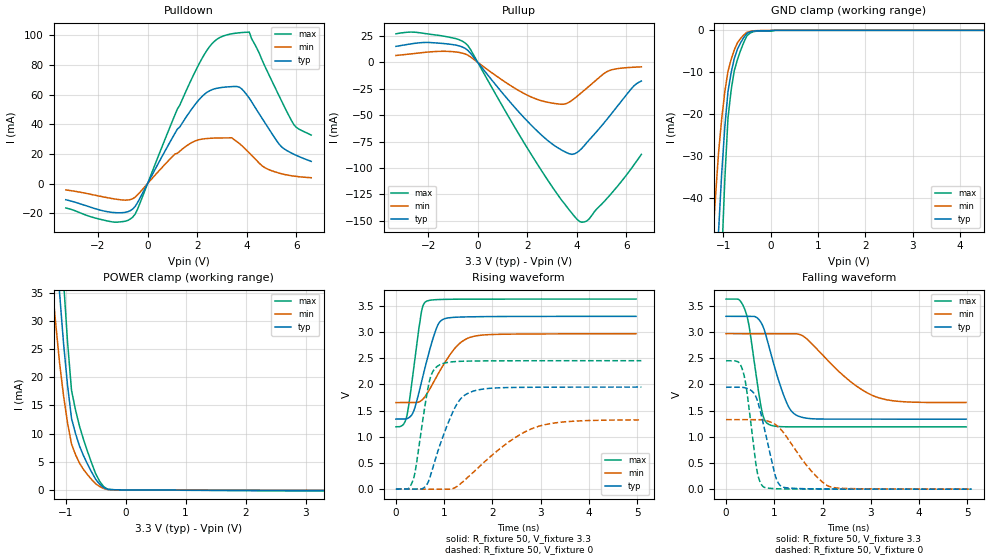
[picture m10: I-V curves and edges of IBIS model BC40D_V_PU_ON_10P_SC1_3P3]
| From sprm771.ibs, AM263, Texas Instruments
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|   Model Cell BC40D_V_PU_ON_10P_SC1_3P3
|BC40D_V_PU_ON_10P_SC1_3P3
[Model]   BC40D_V_PU_ON_10P_SC1_3P3
Model_type   I/O
Polarity   Non-Inverting
Enable   Active-Low
Vinl =  0.8V
Vinh =  2V
Cref =  15pF
Rref =  100.0000M
Vref =  0V
Vmeas =  1.65
C_comp   2.059994p   1.912853p   2.135747p
|[Input load] weak_pu_on
|[Output drive] slow
|[supplytol] 10
|[temp] ind
[Model Spec]
Vinl   0.8V   0.8V   0.8V
Vinh   2V   2V   2V
[Temperature Range]   25   125   -40
[Voltage Range]   3.3   2.97   3.63
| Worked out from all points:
|   slope of the pulldown table from 0 to 0.495 V, typ, clamps not added: 31.8 ohm
|   slope of the pullup table from 0 to 0.495 V, typ, clamps not added: 33.8 ohm
|   GND clamp passes 1 mA (typ) near -0.52 V on its own axis
|   POWER clamp passes 1 mA (typ) near -0.43 V on its own axis
|   rising waveform, R_fixture 50, V_fixture 3.3: 20-80 % time 333ps typ, 531ps min, 208ps max; typ from 1.34 V to 3.3 V
|   rising waveform, R_fixture 50, V_fixture 0: 20-80 % time 466ps typ, 1.07ns min, 244ps max; typ from 0 V to 1.95 V
|   falling waveform, R_fixture 50, V_fixture 3.3: 20-80 % time 385ps typ, 931ps min, 233ps max; typ from 3.3 V to 1.34 V
|   falling waveform, R_fixture 50, V_fixture 0: 20-80 % time 293ps typ, 644ps min, 201ps max; typ from 1.95 V to 0.002 V
| Nom Voltages:
|   VDD=1.1001, VDDS=3.3, VDDS18=1.8, ESD_BIASFET=0, VSS=0, VSSS=0
| Min Voltages:
|   VDD=0.99, VDDS=2.97, VDDS18=1.62, ESD_BIASFET=0, VSS=0, VSSS=0
| Max Voltages:
|   VDD=1.21, VDDS=3.63, VDDS18=1.98, ESD_BIASFET=0, VSS=0, VSSS=0
[POWER_clamp]
|   voltage   I(typ)   I(min)   I(max)
-3.3V     446.9mA    419.5mA    603.9mA
-1.233V   56.55mA    37.52mA    80.26mA
-1.167V   45.63mA    29.9mA     65.05mA
-1.1V     35.1mA     22.66mA    50.24mA
-1.033V   26.08mA    16.76mA    37.18mA
-966.7mV  18.62mA    11.92mA    26.33mA
-900mV    12.7mA     8.149mA    17.69mA
-833.3mV  10mA       6.265mA    14.21mA
-766.7mV  7.795mA    4.753mA    11.3mA
-566.7mV  3.199mA    1.871mA    4.823mA
-366.7mV  433.5uA    268.4uA    618.3uA
3.3V      -100.3uA   -83.23uA   -188.3uA
[Pulldown]
|   voltage   I(typ)   I(min)   I(max)
-3.3V     -10.93mA   -4.311mA   -16.48mA
-1.4V     -19.53mA   -10.23mA   -25.96mA
-600mV    -17.23mA   -10.26mA   -22.66mA
1.1V      33.82mA    19.89mA    46.25mA
2V        55.14mA    29.24mA    78.29mA
2.6V      63.35mA    30.61mA    94.45mA
3.2V      65.21mA    30.81mA    100.4mA
3.7V      65.09mA    27.02mA    101.8mA
4.1V      57.63mA    20.71mA    102.2mA
5.3V      26.68mA    7.058mA    59.31mA
5.9V      19.77mA    5.007mA    39.76mA
6.6V      14.97mA    3.923mA    32.7mA
[Pullup]
|   voltage   I(typ)   I(min)   I(max)
-3.3V     15.12mA    6.498mA    27.02mA
-1.9V     18.73mA    9.943mA    26.53mA
-900mV    16.4mA     9.888mA    22.58mA
-400mV    11.39mA    6.786mA    15.98mA
2.4V      -65.08mA   -35.06mA   -96.18mA
3.5V      -84.52mA   -39.53mA   -134mA
3.8V      -87.17mA   -36.01mA   -143mA
4.1V      -83.7mA    -30.35mA   -150.6mA
4.4V      -75.99mA   -24.42mA   -150.3mA
5.3V      -51.41mA   -7.872mA   -126.6mA
6.3V      -22.29mA   -4.606mA   -97.15mA
6.6V      -17.71mA   -4.277mA   -87.2mA
[GND_clamp]
|   voltage   I(typ)   I(min)   I(max)
-3.3V     -787.2mA   -607.8mA   -1.235A
-1.233V   -85.67mA   -52.14mA   -138.8mA
-1.167V   -66.48mA   -40.37mA   -107.8mA
-1.1V     -48.26mA   -29.37mA   -78.02mA
-1.033V   -34.3mA    -21.2mA    -54.63mA
-966.7mV  -23.1mA    -14.67mA   -35.61mA
-900mV    -14.66mA   -9.802mA   -20.96mA
-833.3mV  -10.12mA   -6.954mA   -14.3mA
-700mV    -4.501mA   -2.964mA   -6.982mA
-500mV    -717.7uA   -486.4uA   -1.28mA
100mV     0A         0A         0A
6.6V      0A         0A         0A
[Ramp]
| variable   typ   min   max
dV/dt_f  1.1795005/0.38538156n 0.79412542/0.93863952n  1.4659129/0.23394861n
dV/dt_r  1.1738038/0.46664111n 0.80280986/1.0806094n  1.4758979/0.24442591n
R_load = 50
[Rising Waveform]
R_fixture = 50
V_fixture = 3.3
V_fixture_min = 2.97
V_fixture_max = 3.63
|   time   V(typ)   V(min)   V(max)
0s        1.338V     1.653V     1.191V
223.4ps   1.344V     1.653V     1.387V
365.8ps   1.486V     1.653V     2.289V
518.6ps   2.003V     1.686V     3.336V
629.4ps   2.417V     1.804V     3.586V
811.6ps   3.001V     2.095V     3.618V
922.1ps   3.207V     2.278V     3.622V
1.255ns   3.284V     2.726V     3.627V
1.553ns   3.291V     2.904V     3.628V
4.974ns   3.3V       2.968V     3.63V
[Rising Waveform]
R_fixture = 50
V_fixture = 0
V_fixture_min = 0
V_fixture_max = 0
|   time   V(typ)   V(min)   V(max)
0s        0V         0V         3.086mV
249.1ps   0V         0V         3.086mV
353.3ps   0V         0V         169.3mV
563.4ps   16.04mV    0V         1.363V
689.9ps   185.6mV    0V         2.047V
905.3ps   826.1mV    0V         2.374V
1.273ns   1.64V      56.7mV     2.439V
1.62ns    1.876V     337.7mV    2.447V
2.935ns   1.947V     1.195V     2.452V
5.085ns   1.949V     1.323V     2.453V
[Falling Waveform]
R_fixture = 50
V_fixture = 3.3
V_fixture_min = 2.97
V_fixture_max = 3.63
|   time   V(typ)   V(min)   V(max)
0s        3.3V       2.969V     3.629V
269.8ps   3.3V       2.969V     3.617V
406ps     3.3V       2.969V     3.388V
482.4ps   3.3V       2.969V     3.083V
737.7ps   3.161V     2.969V     1.514V
887.2ps   2.732V     2.969V     1.238V
1.254ns   1.654V     2.969V     1.192V
1.51ns    1.391V     2.958V     1.191V
3.071ns   1.338V     1.776V     1.19V
4.974ns   1.338V     1.656V     1.19V
[Falling Waveform]
R_fixture = 50
V_fixture = 0
V_fixture_min = 0
V_fixture_max = 0
|   time   V(typ)   V(min)   V(max)
0s        1.948V     1.329V     2.452V
248.7ps   1.948V     1.329V     2.431V
352.3ps   1.943V     1.329V     2.247V
431.2ps   1.926V     1.329V     1.869V
638.8ps   1.719V     1.329V     366mV
786.2ps   1.194V     1.319V     40.36mV
1.029ns   233.9mV    1.231V     10.46mV
1.18ns    41.6mV     1.092V     6.888mV
2.164ns   5.466mV    45.47mV    3.232mV
5.085ns   2.107mV    3.256mV    3.054mV
